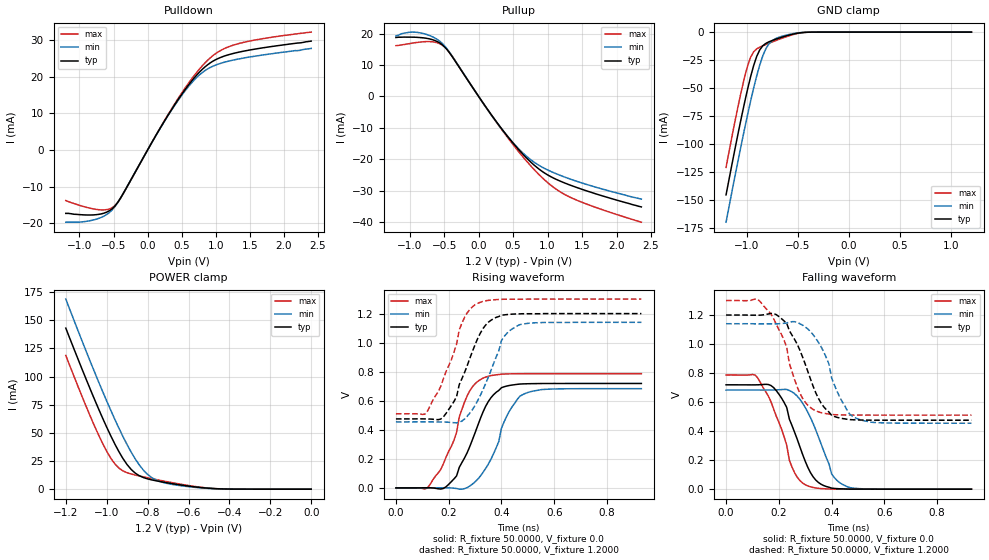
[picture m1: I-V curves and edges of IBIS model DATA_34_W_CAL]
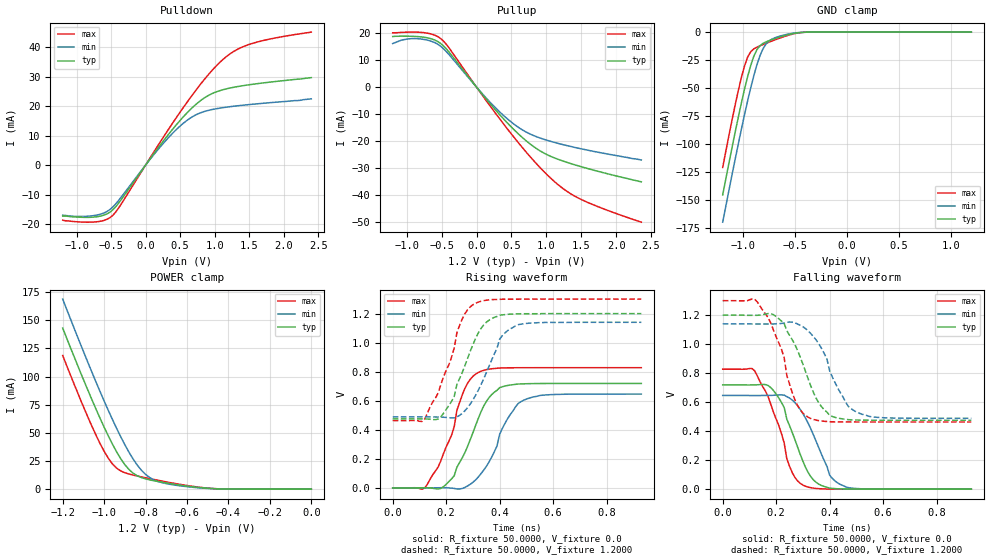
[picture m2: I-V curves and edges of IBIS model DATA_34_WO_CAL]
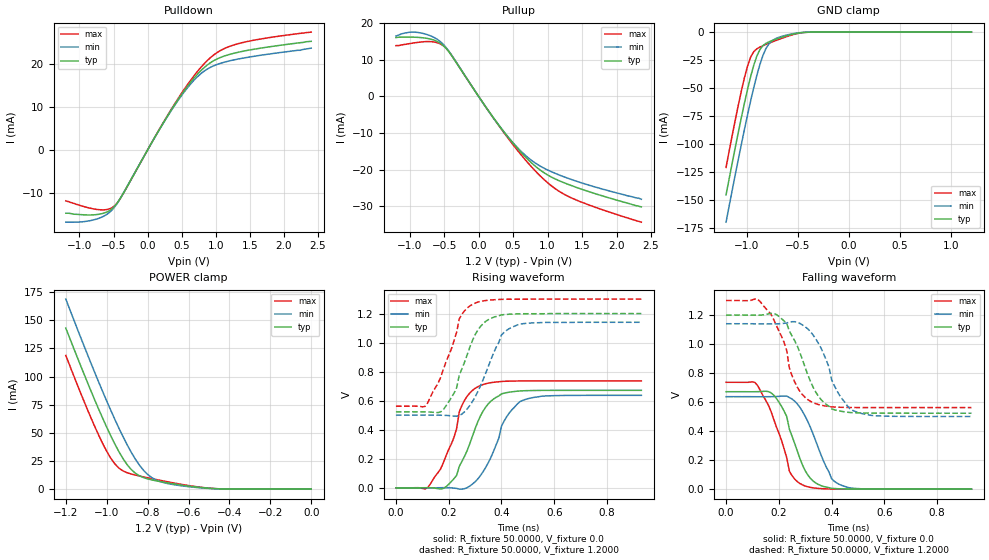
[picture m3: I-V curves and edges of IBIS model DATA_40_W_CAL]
| IBIS file uksl25616ai.ibs created by s2ibis3 verion 3.2
| North Carolina State University, ERL, 2006
| This Model is valid for  Temperature Range -40C<=Tc<=85C
| Valid for LPDDR2-333/400/533/667/800/933/1066 operation
| Part Number   VDD2/VDDQ   Package   Architecture
| SCB4BL256160AFL19GI  1.2 +0.1/-0.06V   FBGA-162   16Meg x 16
[IBIS Ver]   3.2
[File name]  usssl25616ai.ibs
[File Rev]   1.1
[Date]   2022-02-17
[Source]   Simulation of a silicon level SPICE model
[Notes]   IBIS Characteristics for I/O Buffer
   IBIS Model Revision History:
Rev 1.0: 2018-01-17
   - IBIS model file initial creation
Rev 1.1: 2022-02-17
   - add pkg rlc
[disclaimer] The IBIS models are for modeling purpose only and are
   subject to change without any notice. UniIC is not
   responsible for any problems the models may cause.
[Copyright]  Copyright 2022 UniIC Semiconductors Corp. All rights reserved
|   Component SCB4BL256160AFL19GI (FBGA-162, x16)
[Component]   SCB4BL256160AFL19GI
[Manufacturer]  UniIC Semiconductors Corp.
[Package]
|Variable   typ   min   max
R_pkg   0.556   0.378   0.679
L_pkg   1.908nH   1.302nH   2.216nH
C_pkg   0.582pF   0.372pF   0.754pF
[Pin]   signal_name   model_name   R_pin   L_pin   C_pin
E5	VDD2		POWER		NA		NA		NA
E6	VDD1		POWER		NA		NA		NA
F1	VDD1		POWER		NA		NA		NA
F2	VSS		GND		NA		NA		NA
F5	VSS		GND		NA		NA		NA
F6	VSSQ		GND		NA		NA		NA
F7	VDDQ		POWER		NA		NA		NA
F9	VSSQ		GND		NA		NA		NA
F10	VDDQ		POWER		NA		NA		NA
G1	VSS		GND		NA		NA		NA
G2	VDD2		POWER		NA		NA		NA
G3	ZQ0		NC
G5	VDDQ		POWER		NA		NA		NA
G10	VSSQ		GND		NA		NA		NA
H1	VSS		GND		NA		NA		NA
H2	CA9		CLKCA_RCV	0.474		1.978nH		0.453pF
H3	CA8		CLKCA_RCV	0.460		1.859nH		0.433pF
H8	DQ15		DQ		0.640		2.088nH		0.676pF
H9	VDDQ		POWER		NA		NA		NA
H10	VSSQ		GND		NA		NA		NA
J1	VDDCA		POWER		NA		NA		NA
J2	CA6		CLKCA_RCV	0.471		1.976nH		0.469pF
J3	CA7		CLKCA_RCV	0.458		1.961nH		0.412pF
J5	VSSQ		GND		NA		NA		NA
J6	DQ11		DQ		0.620		1.893nH		0.688pF
J7	DQ13		DQ		0.643		2.053nH		0.667pF
J8	DQ14		DQ		0.633		2.077nH		0.656pF
J9	DQ12		DQ		0.592		1.879nH		0.569pF
J10	VDDQ		POWER		NA		NA		NA
K1	VDD2		POWER		NA		NA		NA
K2	CA5		CLKCA_RCV	0.464		1.759nH		0.443pF
K3	VrefCA		NC
K5	DQS1_c		DQ		0.679		2.216nH		0.754pF
K6	DQS1_t		DQ		0.674		2.149nH		0.750pF
K7	DQ10		DQ		0.597		1.926nH		0.614pF
K8	DQ9		DQ		0.587		1.830nH		0.662pF
K9	DQ8		DQ		0.579		1.883nH		0.630pF
K10	VSSQ		GND		NA		NA		NA
L1	VDDCA		POWER		NA		NA		NA
L2	VSS		GND		NA		NA		NA
L3	CK_c		CLKCA_RCV	0.378		1.454nH		0.372pF
L5	DM1		DQ		0.651		1.935nH		0.742pF
L6	VDDQ		POWER		NA		NA		NA
M1	VSS		GND		NA		NA		NA
M3	CK_t		CLKCA_RCV	0.389		1.302nH		0.400pF
M5	VSSQ		GND		NA		NA		NA
M6	VDDQ		POWER		NA		NA		NA
M7	VDD2		POWER		NA		NA		NA
M8	VSS		GND		NA		NA		NA
M9	VrefDQ		NC
N1	CKE		CLKCA_RCV	0.446		1.614nH		0.442pF
N5	DM0		DQ		0.641		1.892nH		0.746pF
N6	VDDQ		POWER		NA		NA		NA
P1	CS_n		CLKCA_RCV	0.447		1.842nH		0.456pF
P5	DQS0_c		DQ		0.648		2.065nH		0.741pF
P6	DQS0_t		DQ		0.647		2.022nH		0.742pF
P7	DQ5		DQ		0.600		2.057nH		0.612pF
P8	DQ6		DQ		0.585		1.896nH		0.623pF
P9	DQ7		DQ		0.578		1.887nH		0.582pF
P10	VSSQ		GND		NA		NA		NA
R1	CA4		CLKCA_RCV	0.464		1.944nH		0.462pF
R2	CA3		CLKCA_RCV	0.448		2.047nH		0.405pF
R3	CA2		CLKCA_RCV	0.448		1.881nH		0.471pF
R5	VSSQ		GND		NA		NA		NA
R6	DQ4		DQ		0.623		1.911nH		0.703pF
R7	DQ2		DQ		0.641		1.973nH		0.688pF
R8	DQ1		DQ		0.632		2.051nH		0.649pF
R9	DQ3		DQ		0.598		1.884nH		0.594pF
R10	VDDQ		POWER		NA		NA		NA
T1	VSS		GND		NA		NA		NA
T2	VDDCA		POWER		NA		NA		NA
T3	CA1		CLKCA_RCV	0.470		1.857nH		0.486pF
T8	DQ0		DQ		0.629		2.028nH		0.661pF
T9	VDDQ		POWER		NA		NA		NA
T10	VSSQ		GND		NA		NA		NA
U1	VSS		GND		NA		NA		NA
U2	VDD2		POWER		NA		NA		NA
U3	CA0		CLKCA_RCV	0.487		1.606nH		0.509pF
U5	VDDQ		POWER		NA		NA		NA
U10	VSSQ		GND		NA		NA		NA
V1	VDD1		POWER		NA		NA		NA
V2	VSS		GND		NA		NA		NA
V5	VSS		GND		NA		NA		NA
V6	VSSQ		GND		NA		NA		NA
V7	VDDQ		POWER		NA		NA		NA
V9	VSSQ		GND		NA		NA		NA
V10	VDDQ		POWER		NA		NA		NA
W5	VDD2		POWER		NA		NA		NA
W6	VDD1		POWER		NA		NA		NA
|*****************************  Diff Pin  *************************************
[Diff Pin]  inv_pin  vdiff   tdelay_typ  tdelay_min  tdelay_max
M3   L3   0.44000V   NA   NA   NA
P6   P5   0.44000V   NA   NA   NA
K6   K5   0.44000V   NA   NA   NA
|*****************************  Model Selector ********************************
[Model Selector]   DQ
DATA_34_W_CAL   RZQ/7 Output Driver, With ZQ Cal
DATA_40_W_CAL   RZQ/6 Output Driver, With ZQ Cal
DATA_48_W_CAL   RZQ/5 Output Driver, With ZQ Cal
DATA_60_W_CAL   RZQ/4 Output Driver, With ZQ Cal
DATA_80_W_CAL   RZQ/3 Output Driver, With ZQ Cal
DATA_120_W_CAL   RZQ/2 Output Driver, With ZQ Cal
DATA_34_WO_CAL   RZQ/7 Output Driver, Without ZQ Cal
DATA_40_WO_CAL   RZQ/6 Output Driver, Without ZQ Cal
DATA_48_WO_CAL   RZQ/5 Output Driver, Without ZQ Cal
DATA_60_WO_CAL   RZQ/4 Output Driver, Without ZQ Cal
DATA_80_WO_CAL   RZQ/3 Output Driver, Without ZQ Cal
DATA_120_WO_CAL   RZQ/2 Output Driver, Without ZQ Cal
DATA_RCV   Data/Data Strobe/Data Mask Receiver
| Models and submodels in the file (14): DATA_34_W_CAL (I/O), DATA_34_WO_CAL (I/O), DATA_40_W_CAL (I/O), DATA_40_WO_CAL (I/O), DATA_48_W_CAL (I/O), DATA_48_WO_CAL (I/O), DATA_60_W_CAL (I/O), DATA_60_WO_CAL (I/O), DATA_80_W_CAL (I/O), DATA_80_WO_CAL (I/O), DATA_120_W_CAL (I/O), DATA_120_WO_CAL (I/O), DATA_RCV (Input), CLKCA_RCV (Input)
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|   Model DATA_34_W_CAL
[Model]  DATA_34_W_CAL
Model_type I/O
Polarity   Non-Inverting
Enable   Active-High
Vinl =   0.3800V
Vinh =   0.8200V
Vmeas =  0.6000V
Cref =   5.0000pF
Rref =   50.0000
Vref =   0.6000V
C_comp   1.7430pF   1.7110pF   1.7640pF
[Temperature Range]   25.0000   85.0000   -40.0000
[Voltage Range]   1.2000V   1.1400V   1.3000V
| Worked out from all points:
|   slope of the pulldown table from 0 to 0.18 V, typ, clamps not added: 31 ohm
|   slope of the pullup table from 0 to 0.18 V, typ, clamps not added: 31.6 ohm
|   GND clamp passes 1 mA (typ) near -0.50 V on its own axis
|   POWER clamp passes 1 mA (typ) near -0.51 V on its own axis
|   rising waveform, R_fixture 50.0000, V_fixture 0.0: 20-80 % time 103ps typ, 95.3ps min, 91.3ps max; typ from 0 V to 0.719 V
|   rising waveform, R_fixture 50.0000, V_fixture 1.2000: 20-80 % time 89.8ps typ, 91.2ps min, 90.2ps max; typ from 0.475 V to 1.2 V
|   falling waveform, R_fixture 50.0000, V_fixture 0.0: 20-80 % time 85.3ps typ, 90.5ps min, 85.5ps max; typ from 0.719 V to 0 V
|   falling waveform, R_fixture 50.0000, V_fixture 1.2000: 20-80 % time 99.7ps typ, 90.8ps min, 89.4ps max; typ from 1.2 V to 0.475 V
[Pulldown]
|Voltage   I(typ)   I(min)   I(max)
-1.2V     -17.3mA    -19.7mA    -13.8mA
-760mV    -17.66mA   -18.92mA   -16.19mA
-600mV    -16.96mA   -17.61mA   -16.27mA
-480mV    -15.3mA    -15.47mA   -15.18mA
-360mV    -11.96mA   -11.94mA   -12.01mA
80mV      2.621mA    2.599mA    2.653mA
360mV     11.26mA    11.11mA    11.47mA
640mV     18.67mA    18.19mA    19.23mA
840mV     22.64mA    21.63mA    23.72mA
1.04V     25mA       23.45mA    26.81mA
1.28V     26.44mA    24.62mA    28.73mA
2.4V      29.7mA     27.7mA     32.16mA
[Pullup]
|Voltage   I(typ)   I(min)   I(max)
-1.2V     18.8mA     19.3mA     16.2mA
-1V       18.92mA    20.49mA    16.86mA
-800mV    18.69mA    20.06mA    17.45mA
-600mV    17.51mA    18.18mA    17.13mA
-480mV    15.5mA     15.77mA    15.52mA
80mV      -2.576mA   -2.617mA   -2.601mA
360mV     -11.05mA   -11.07mA   -11.3mA
600mV     -17.41mA   -17.1mA    -18.12mA
840mV     -22.52mA   -21.46mA   -24.1mA
1.08V     -25.94mA   -24.21mA   -28.86mA
1.32V     -28.19mA   -26.26mA   -32.04mA
2.36V     -35.2mA    -32.7mA    -40.07mA
[GND_clamp]
|Voltage   I(typ)   I(min)   I(max)
-1.2V     -145.3mA   -169.7mA   -120.8mA
-1.11V    -103.1mA   -127.3mA   -78.51mA
-1.05V    -76.2mA    -100.1mA   -52.43mA
-990mV    -51.2mA    -74mA      -30.39mA
-960mV    -39.9mA    -61.63mA   -22.48mA
-900mV    -21.67mA   -39mA      -15mA
-870mV    -15.78mA   -29.25mA   -13.45mA
-810mV    -10.04mA   -14.72mA   -11.07mA
-750mV    -7.557mA   -7.71mA    -8.865mA
-600mV    -3.111mA   -2.463mA   -3.804mA
-420mV    -215.4uA   -156.1uA   -235uA
1.2V      1.597nA    5.589nA    1.463nA
[POWER_clamp]
|Voltage   I(typ)   I(min)   I(max)
-1.2V     143mA      168.8mA    118.7mA
-1.06V    79.88mA    104.3mA    56.26mA
-1.02V    63.08mA    86.79mA    40.63mA
-980mV    47.32mA    69.97mA    27.48mA
-940mV    33.2mA     54.05mA    18.67mA
-880mV    17.43mA    32.78mA    13.45mA
-840mV    11.87mA    21.34mA    11.69mA
-800mV    9.133mA    13.1mA     10.12mA
-720mV    6.135mA    5.731mA    7.166mA
-560mV    1.838mA    1.456mA    2.161mA
-420mV    156.9uA    132.7uA    153uA
0V        1.597nA    1.927nA    2.16nA
[Ramp]
| variable   typ   min   max
dV/dt_r  0.4314/96.1802p   0.4099/97.9167p   0.4720/94.2430p
dV/dt_f  0.4350/92.7485p   0.4113/93.7685p   0.4739/92.4509p
R_load = 50.0000
[Rising Waveform]
R_fixture= 50.0000
V_fixture= 0.0
V_fixture_min= 0.0
V_fixture_max= 0.0
|time   V(typ)   V(min)   V(max)
0s        0V         0V         0V
120ps     1.003mV    167.7uV    1.23mV
190ps     8.093mV    1.271mV    212mV
230ps     83.25mV    -3.9mV     383.2mV
270ps     242.6mV    2.235mV    634.2mV
330ps     522.8mV    107mV      755.5mV
380ps     658.4mV    277mV      778.6mV
400ps     690mV      411.9mV    783.1mV
480ps     715.9mV    641.8mV    786.4mV
930ps     719mV      683.2mV    786.7mV
[Rising Waveform]
R_fixture= 50.0000
V_fixture= 1.2000
V_fixture_min= 1.1400
V_fixture_max= 1.3000
|time   V(typ)   V(min)   V(max)
0s        475mV      454.5mV    510.1mV
110ps     475mV      454.7mV    507.6mV
180ps     489.3mV    453.7mV    751.9mV
230ps     629.5mV    447.9mV    991.9mV
260ps     794.2mV    474.4mV    1.174V
310ps     1.029V     601.4mV    1.271V
350ps     1.14V      762mV      1.291V
400ps     1.189V     1.015V     1.298V
460ps     1.198V     1.116V     1.299V
930ps     1.2V       1.14V      1.3V
[Falling Waveform]
R_fixture= 50.0000
V_fixture= 0.0
V_fixture_min= 0.0
V_fixture_max= 0.0
|time   V(typ)   V(min)   V(max)
0s        719mV      683.2mV    786.7mV
110ps     718.8mV    683mV      786.5mV
180ps     700.3mV    683.4mV    553.5mV
230ps     562.6mV    687.2mV    302.3mV
250ps     437.6mV    670.6mV    151.9mV
310ps     150mV      529.8mV    22.24mV
350ps     46.23mV    360.6mV    5.968mV
400ps     7.106mV    105.5mV    822.2uV
460ps     926.8uV    16.43mV    95.79uV
930ps     0V         0V         0V
[Falling Waveform]
R_fixture= 50.0000
V_fixture= 1.2000
V_fixture_min= 1.1400
V_fixture_max= 1.3000
|time   V(typ)   V(min)   V(max)
0s        1.2V       1.14V      1.3V
120ps     1.199V     1.139V     1.308V
210ps     1.175V     1.141V     1.066V
280ps     956.7mV    1.14V      660.1mV
340ps     664mV      1.039V     540.2mV
390ps     531.3mV    861.7mV    517.7mV
400ps     508.8mV    767.4mV    514.4mV
460ps     481.3mV    539.8mV    510.8mV
490ps     477.5mV    491.6mV    510.4mV
930ps     475mV      454.5mV    510.1mV
|   Model DATA_34_WO_CAL
[Model]  DATA_34_WO_CAL
Model_type I/O
Polarity   Non-Inverting
Enable   Active-High
Vinl =   0.3800V
Vinh =   0.8200V
Vmeas =  0.6000V
Cref =   5.0000pF
Rref =   50.0000
Vref =   0.6000V
C_comp   1.7430pF   1.7110pF   1.7640pF
[Temperature Range]   25.0000   85.0000   -40.0000
[Voltage Range]   1.2000V   1.1400V   1.3000V
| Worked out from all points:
|   slope of the pulldown table from 0 to 0.18 V, typ, clamps not added: 31 ohm
|   slope of the pullup table from 0 to 0.18 V, typ, clamps not added: 31.6 ohm
|   GND clamp passes 1 mA (typ) near -0.50 V on its own axis
|   POWER clamp passes 1 mA (typ) near -0.51 V on its own axis
|   rising waveform, R_fixture 50.0000, V_fixture 0.0: 20-80 % time 103ps typ, 102ps min, 89.8ps max; typ from 0 V to 0.719 V
|   rising waveform, R_fixture 50.0000, V_fixture 1.2000: 20-80 % time 89.8ps typ, 93.5ps min, 89.9ps max; typ from 0.475 V to 1.2 V
|   falling waveform, R_fixture 50.0000, V_fixture 0.0: 20-80 % time 85.3ps typ, 93.4ps min, 84.8ps max; typ from 0.719 V to 0 V
|   falling waveform, R_fixture 50.0000, V_fixture 1.2000: 20-80 % time 99.7ps typ, 97.9ps min, 84.6ps max; typ from 1.2 V to 0.475 V
[Pulldown]
|Voltage   I(typ)   I(min)   I(max)
-1.2V     -17.3mA    -17mA      -18.7mA
-720mV    -17.57mA   -17.03mA   -19.27mA
-480mV    -15.3mA    -14.35mA   -17.17mA
-360mV    -11.96mA   -11.09mA   -13.5mA
200mV     6.437mA    5.837mA    7.408mA
520mV     15.7mA     13.68mA    18.66mA
680mV     19.58mA    16.44mA    23.9mA
840mV     22.64mA    18.12mA    28.77mA
1.2V      26.05mA    19.77mA    37.38mA
1.4V      26.93mA    20.31mA    40.08mA
1.6V      27.6mA     20.77mA    41.68mA
2.4V      29.7mA     22.5mA     45.16mA
[Pullup]
|Voltage   I(typ)   I(min)   I(max)
-1.2V     18.8mA     16.2mA     20.2mA
-1.04V    18.92mA    17.64mA    20.38mA
-840mV    18.77mA    17.99mA    20.41mA
-640mV    17.89mA    16.97mA    19.68mA
-520mV    16.35mA    15.32mA    18.19mA
-400mV    13.24mA    12.29mA    14.79mA
320mV     -9.896mA   -8.925mA   -11.39mA
600mV     -17.41mA   -14.96mA   -20.69mA
840mV     -22.52mA   -18.25mA   -27.96mA
1.12V     -26.37mA   -20.59mA   -35.21mA
1.4V      -28.83mA   -22.38mA   -40.43mA
2.36V     -35.2mA    -27.1mA    -50.22mA
[GND_clamp]
|Voltage   I(typ)   I(min)   I(max)
-1.2V     -145.3mA   -169.7mA   -120.8mA
-1.11V    -103.1mA   -127.3mA   -78.51mA
-1.05V    -76.2mA    -100.1mA   -52.43mA
-990mV    -51.2mA    -74mA      -30.39mA
-960mV    -39.9mA    -61.63mA   -22.48mA
-900mV    -21.67mA   -39mA      -15mA
-870mV    -15.78mA   -29.25mA   -13.45mA
-810mV    -10.04mA   -14.72mA   -11.07mA
-750mV    -7.557mA   -7.71mA    -8.865mA
-600mV    -3.111mA   -2.463mA   -3.804mA
-420mV    -215.4uA   -156.1uA   -235uA
1.2V      1.597nA    5.589nA    1.463nA
[POWER_clamp]
|Voltage   I(typ)   I(min)   I(max)
-1.2V     143mA      168.8mA    118.7mA
-1.06V    79.88mA    104.3mA    56.26mA
-1.02V    63.08mA    86.79mA    40.63mA
-980mV    47.32mA    69.97mA    27.48mA
-940mV    33.2mA     54.05mA    18.67mA
-880mV    17.43mA    32.78mA    13.45mA
-840mV    11.87mA    21.34mA    11.69mA
-800mV    9.133mA    13.1mA     10.12mA
-720mV    6.135mA    5.731mA    7.166mA
-560mV    1.838mA    1.456mA    2.161mA
-420mV    156.9uA    132.7uA    153uA
0V        1.597nA    1.927nA    2.16nA
[Ramp]
| variable   typ   min   max
dV/dt_r  0.4314/96.1802p   0.3877/0.1037n   0.4965/92.7944p
dV/dt_f  0.4350/92.7485p   0.3908/0.1023n   0.5020/88.0000p
R_load = 50.0000
[Rising Waveform]
R_fixture= 50.0000
V_fixture= 0.0
V_fixture_min= 0.0
V_fixture_max= 0.0
|time   V(typ)   V(min)   V(max)
0s        0V         0V         0V
120ps     1.003mV    167.6uV    141.1uV
180ps     -3.556mV   1.175mV    185.9mV
230ps     83.25mV    -3.578mV   420.7mV
270ps     242.6mV    3.012mV    684.9mV
320ps     477.7mV    74.74mV    794.5mV
370ps     641.8mV    211.8mV    820.1mV
400ps     690mV      369.4mV    825.2mV
490ps     716.6mV    603.6mV    827.4mV
930ps     719mV      646.2mV    827.5mV
[Rising Waveform]
R_fixture= 50.0000
V_fixture= 1.2000
V_fixture_min= 1.1400
V_fixture_max= 1.3000
|time   V(typ)   V(min)   V(max)
0s        475mV      488.7mV    463.3mV
110ps     475mV      489mV      457.1mV
180ps     489.3mV    487.1mV    709.4mV
230ps     629.5mV    481.6mV    962.8mV
260ps     794.2mV    513mV      1.163V
310ps     1.029V     637.1mV    1.271V
350ps     1.14V      791.9mV    1.292V
400ps     1.189V     1.024V     1.298V
460ps     1.198V     1.116V     1.299V
930ps     1.2V       1.14V      1.3V
[Falling Waveform]
R_fixture= 50.0000
V_fixture= 0.0
V_fixture_min= 0.0
V_fixture_max= 0.0
|time   V(typ)   V(min)   V(max)
0s        719mV      646.2mV    827.5mV
120ps     719.1mV    645.9mV    814.7mV
170ps     714.5mV    646.3mV    637.9mV
210ps     628.4mV    649.6mV    438.2mV
250ps     437.6mV    628.2mV    157.9mV
300ps     192.5mV    521mV      28.39mV
350ps     46.23mV    327.5mV    4.803mV
400ps     7.106mV    96.75mV    563uV
440ps     2.016mV    32.57mV    133.9uV
930ps     0V         0V         0V
[Falling Waveform]
R_fixture= 50.0000
V_fixture= 1.2000
V_fixture_min= 1.1400
V_fixture_max= 1.3000
|time   V(typ)   V(min)   V(max)
0s        1.2V       1.14V      1.3V
130ps     1.199V     1.139V     1.29V
230ps     1.142V     1.145V     905.3mV
240ps     1.092V     1.151V     783mV
270ps     997.7mV    1.147V     616.5mV
320ps     758.6mV    1.091V     495.9mV
370ps     567.9mV    969.5mV    469.8mV
400ps     508.8mV    815.3mV    465.1mV
500ps     477mV      532.7mV    463.3mV
930ps     475mV      488.7mV    463.3mV
|   Model DATA_40_W_CAL
[Model]  DATA_40_W_CAL
Model_type I/O
Polarity   Non-Inverting
Enable   Active-High
Vinl =   0.3800V
Vinh =   0.8200V
Vmeas =  0.6000V
Cref =   5.0000pF
Rref =   50.0000
Vref =   0.6000V
C_comp   1.7430pF   1.7110pF   1.7640pF
[Temperature Range]   25.0000   85.0000   -40.0000
[Voltage Range]   1.2000V   1.1400V   1.3000V
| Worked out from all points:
|   slope of the pulldown table from 0 to 0.18 V, typ, clamps not added: 36.2 ohm
|   slope of the pullup table from 0 to 0.18 V, typ, clamps not added: 36.7 ohm
|   GND clamp passes 1 mA (typ) near -0.50 V on its own axis
|   POWER clamp passes 1 mA (typ) near -0.51 V on its own axis
|   rising waveform, R_fixture 50.0000, V_fixture 0.0: 20-80 % time 95.4ps typ, 91.7ps min, 82.6ps max; typ from 0 V to 0.672 V
|   rising waveform, R_fixture 50.0000, V_fixture 1.2000: 20-80 % time 81.5ps typ, 91.2ps min, 82.8ps max; typ from 0.523 V to 1.2 V
|   falling waveform, R_fixture 50.0000, V_fixture 0.0: 20-80 % time 77.9ps typ, 89.8ps min, 80.1ps max; typ from 0.672 V to 0 V
|   falling waveform, R_fixture 50.0000, V_fixture 1.2000: 20-80 % time 96.1ps typ, 89.6ps min, 83.4ps max; typ from 1.2 V to 0.523 V
[Pulldown]
|Voltage   I(typ)   I(min)   I(max)
-1.2V     -14.8mA    -16.9mA    -11.9mA
-720mV    -15.06mA   -16.02mA   -13.97mA
-560mV    -14.21mA   -14.62mA   -13.79mA
-480mV    -13.11mA   -13.26mA   -13.01mA
-360mV    -10.25mA   -10.23mA   -10.29mA
80mV      2.246mA    2.228mA    2.274mA
360mV     9.654mA    9.524mA    9.83mA
640mV     16mA       15.59mA    16.49mA
840mV     19.41mA    18.54mA    20.33mA
1.04V     21.43mA    20.1mA     22.98mA
1.28V     22.66mA    21.1mA     24.63mA
2.4V      25.4mA     23.8mA     27.56mA
[Pullup]
|Voltage   I(typ)   I(min)   I(max)
-1.2V     16.1mA     16.5mA     13.9mA
-1V       16.22mA    17.56mA    14.45mA
-840mV    16.09mA    17.37mA    14.89mA
-640mV    15.36mA    16.07mA    14.87mA
-480mV    13.33mA    13.56mA    13.34mA
120mV     -3.305mA   -3.352mA   -3.342mA
360mV     -9.503mA   -9.52mA    -9.721mA
600mV     -14.97mA   -14.7mA    -15.58mA
840mV     -19.35mA   -18.43mA   -20.72mA
1.08V     -22.27mA   -20.77mA   -24.79mA
1.32V     -24.18mA   -22.53mA   -27.5mA
2.36V     -30.2mA    -28.1mA    -34.37mA
[GND_clamp]
|Voltage   I(typ)   I(min)   I(max)
-1.2V     -145.3mA   -169.7mA   -120.8mA
-1.11V    -103.1mA   -127.3mA   -78.51mA
-1.05V    -76.2mA    -100.1mA   -52.43mA
-990mV    -51.2mA    -74mA      -30.39mA
-960mV    -39.9mA    -61.63mA   -22.48mA
-900mV    -21.67mA   -39mA      -15mA
-870mV    -15.78mA   -29.25mA   -13.45mA
-810mV    -10.04mA   -14.72mA   -11.07mA
-750mV    -7.557mA   -7.71mA    -8.865mA
-600mV    -3.111mA   -2.463mA   -3.804mA
-420mV    -215.4uA   -156.1uA   -235uA
1.2V      1.597nA    5.589nA    1.463nA
[POWER_clamp]
|Voltage   I(typ)   I(min)   I(max)
-1.2V     143mA      168.8mA    118.7mA
-1.06V    79.88mA    104.3mA    56.26mA
-1.02V    63.08mA    86.79mA    40.63mA
-980mV    47.32mA    69.97mA    27.48mA
-940mV    33.2mA     54.05mA    18.67mA
-880mV    17.43mA    32.78mA    13.45mA
-840mV    11.87mA    21.34mA    11.69mA
-800mV    9.133mA    13.1mA     10.12mA
-720mV    6.135mA    5.731mA    7.166mA
-560mV    1.838mA    1.456mA    2.161mA
-420mV    156.9uA    132.7uA    153uA
0V        1.597nA    1.927nA    2.16nA
[Ramp]
| variable   typ   min   max
dV/dt_r  0.4030/90.3786p   0.3824/94.5447p   0.4419/86.1430p
dV/dt_f  0.4060/89.3830p   0.3835/92.6339p   0.4427/86.8818p
R_load = 50.0000
[Rising Waveform]
R_fixture= 50.0000
V_fixture= 0.0
V_fixture_min= 0.0
V_fixture_max= 0.0
|time   V(typ)   V(min)   V(max)
0s        0V         0V         0V
120ps     1.042mV    168.2uV    1.036mV
190ps     7.806mV    1.341mV    221.7mV
220ps     63.13mV    -1.868mV   348.2mV
250ps     182mV      -9.011mV   567.3mV
320ps     494mV      83.8mV     704.7mV
360ps     596.9mV    210.1mV    724.4mV
410ps     651.9mV    460.1mV    733.7mV
470ps     667.5mV    593.7mV    736mV
930ps     671.6mV    637.3mV    736.5mV
[Rising Waveform]
R_fixture= 50.0000
V_fixture= 1.2000
V_fixture_min= 1.1400
V_fixture_max= 1.3000
|time   V(typ)   V(min)   V(max)
0s        523.4mV    500.8mV    562.2mV
110ps     523.3mV    501.1mV    560.7mV
180ps     539.9mV    499.7mV    817.8mV
230ps     688.5mV    493.3mV    1.072V
240ps     775.7mV    498.4mV    1.163V
300ps     1.054V     625.7mV    1.272V
340ps     1.146V     788.8mV    1.29V
400ps     1.191V     1.053V     1.298V
440ps     1.196V     1.106V     1.299V
930ps     1.2V       1.14V      1.3V
[Falling Waveform]
R_fixture= 50.0000
V_fixture= 0.0
V_fixture_min= 0.0
V_fixture_max= 0.0
|time   V(typ)   V(min)   V(max)
0s        671.6mV    637.3mV    736.5mV
110ps     671.5mV    637mV      734.5mV
180ps     649.1mV    637.7mV    484.9mV
230ps     500.3mV    641.1mV    216.4mV
240ps     413.2mV    631.4mV    124.1mV
290ps     165mV      534.7mV    29.18mV
330ps     56.08mV    379.4mV    9.051mV
400ps     5.96mV     71.34mV    863.2uV
430ps     2.556mV    32.33mV    356.7uV
930ps     0V         0V         0V
[Falling Waveform]
R_fixture= 50.0000
V_fixture= 1.2000
V_fixture_min= 1.1400
V_fixture_max= 1.3000
|time   V(typ)   V(min)   V(max)
0s        1.2V       1.14V      1.3V
120ps     1.199V     1.139V     1.308V
200ps     1.191V     1.14V      1.091V
230ps     1.141V     1.145V     953.9mV
260ps     1.023V     1.154V     738.7mV
330ps     702.2mV    1.062V     596mV
370ps     598.6mV    931.4mV    575mV
420ps     542.6mV    678.7mV    565.1mV
480ps     527.2mV    543.2mV    562.7mV
930ps     523.4mV    500.8mV    562.2mV
